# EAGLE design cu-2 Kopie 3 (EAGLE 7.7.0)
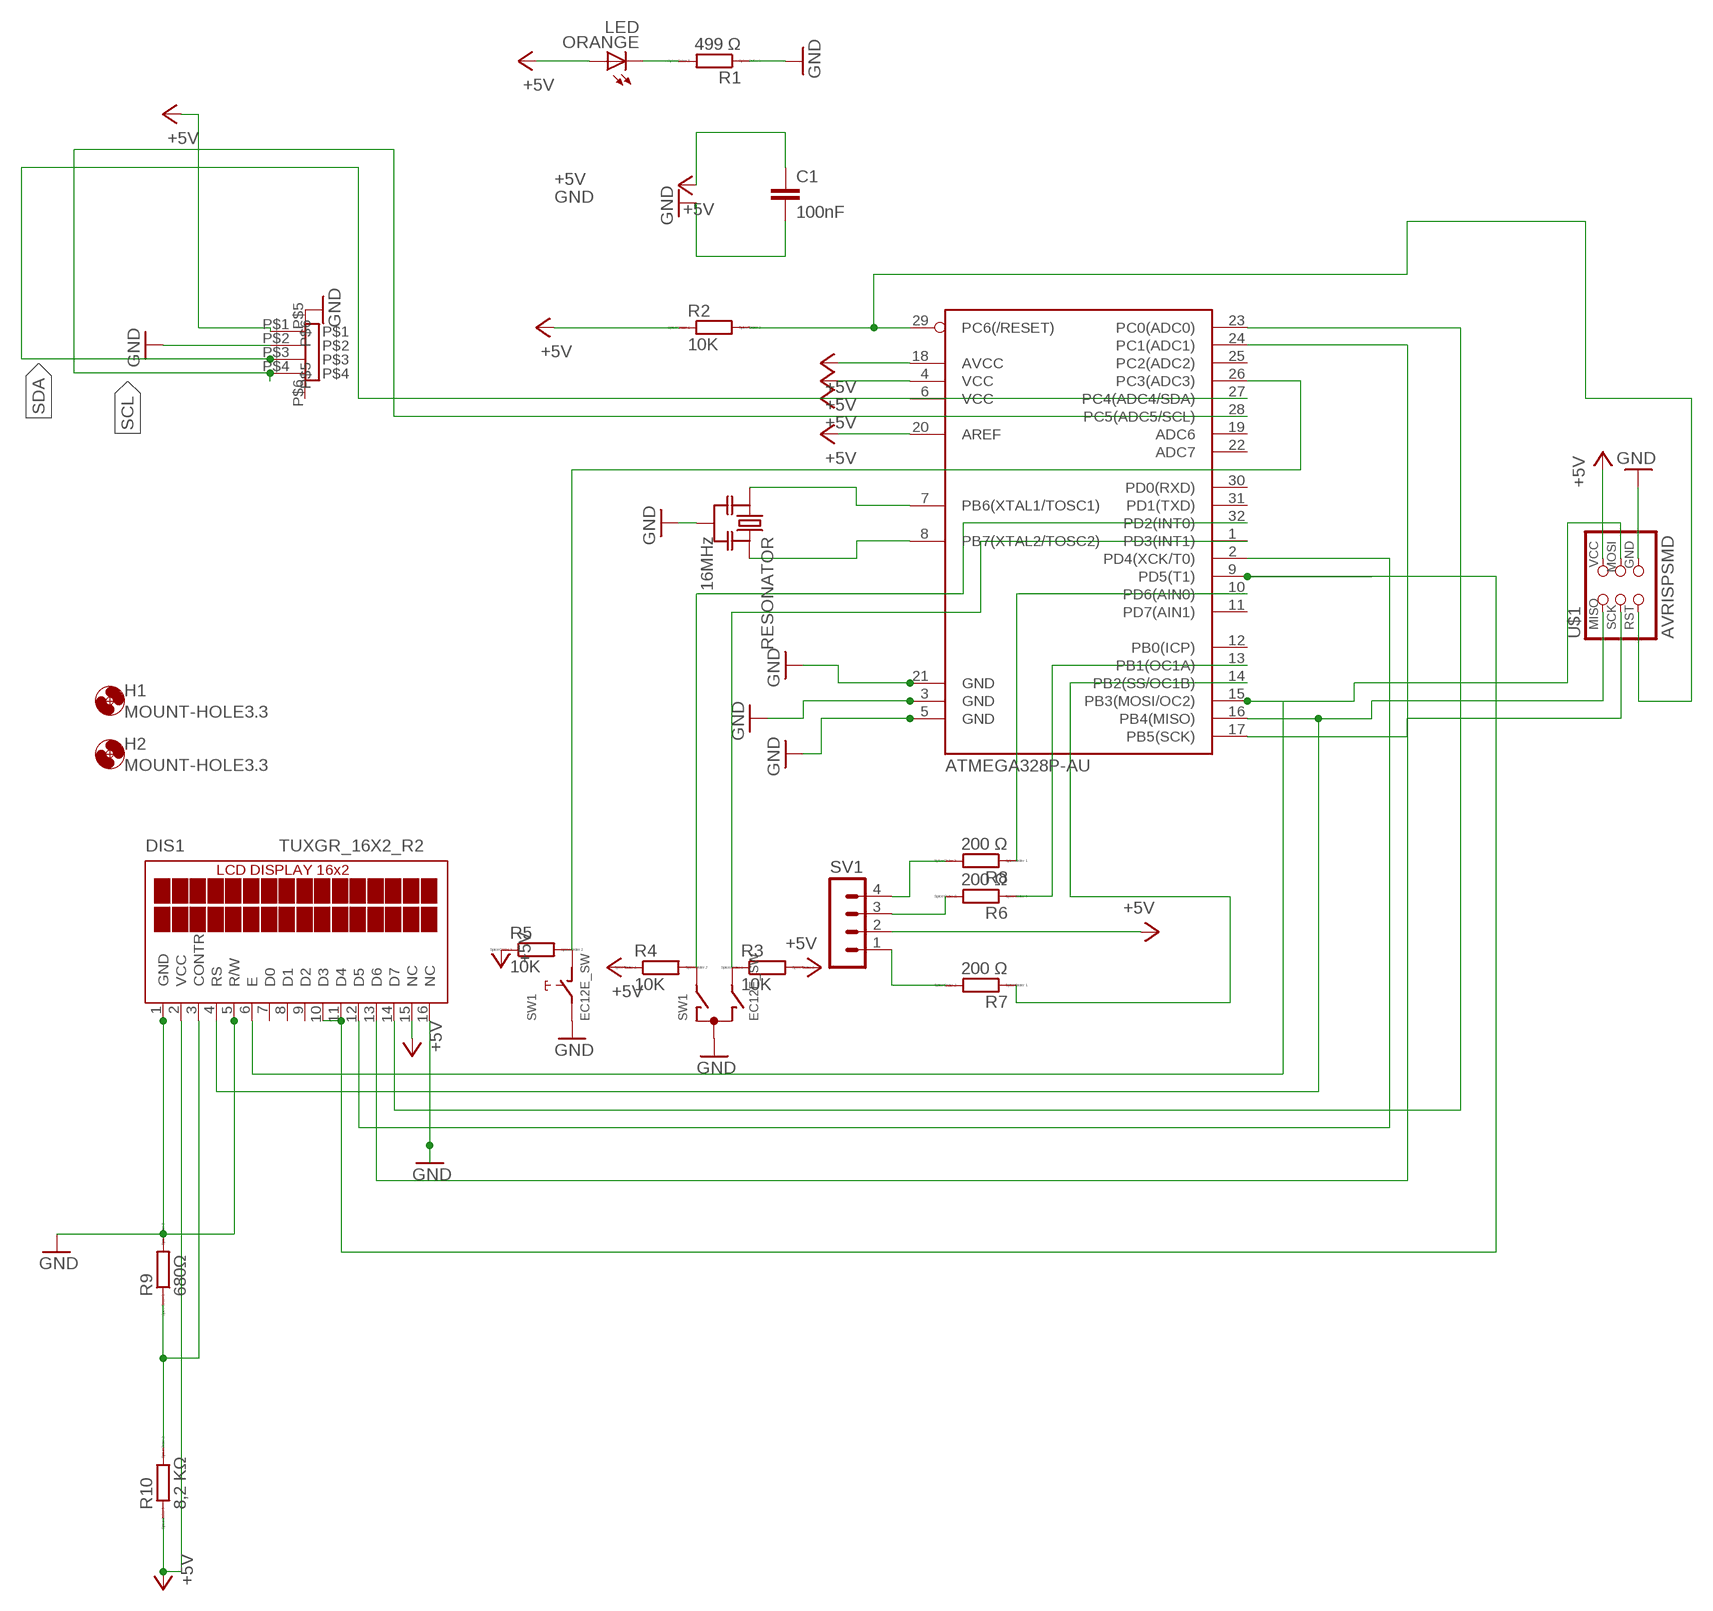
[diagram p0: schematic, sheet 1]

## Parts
ATMEGA328P-AU  ATMEGA88-THIN  [TQFP32-08THIN]
C1  100nF  C-EUC1206  [C1206]
DIS1  TUXGR_16X2_R2  [TUXGR_16X2_R2]
H1  MOUNT-HOLE3.3  [3,3]
H2  MOUNT-HOLE3.3  [3,3]
ORANGE  LED  [LED1206]
R1  499 Ω  RR1206  [R1206]
R2  10K  RR1206  [R1206]
R3  10K  RR1206  [R1206]
R4  10K  RR1206  [R1206]
R5  10K  RR1206  [R1206]
R6  200 Ω  RR1206  [R1206]
R7  200 Ω  RR1206  [R1206]
R8  200 Ω  RR1206  [R1206]
R9  680Ω  RR1206  [R1206]
R10  8,2 KΩ  RR1206  [R1206]
RESONATOR  16MHz  RESONATOR-MURATACSTCR_G  [RESONATOR_MURATA3]
SV1  MA04-1  [MA04-1]
SW1  EC12E_SW  [ALPS_EC12E_SW]
U$1  AVRISPSMD  [2X03SMD]
U$2  PHP4_SM4  [PH4P_SM4]

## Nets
+5V: ATMEGA328P-AU.4(VCC) ATMEGA328P-AU.6(VCC) ATMEGA328P-AU.18(AVCC) ATMEGA328P-AU.20(AREF) C1.1 DIS1.2(VCC) DIS1.15(NC) ORANGE.1(A) R2.1 R3.2 R4.1 R5.1 R10.1 SV1.2 U$1.2(VCC) U$2.P$1
DISP_D4: ATMEGA328P-AU.9(PD5(T1)) DIS1.11(D4)
DISP_D5: ATMEGA328P-AU.2(PD4(XCK/T0)) DIS1.12(D5)
DISP_D6: ATMEGA328P-AU.24(PC1(ADC1)) DIS1.13(D6)
DISP_D7: ATMEGA328P-AU.23(PC0(ADC0)) DIS1.14(D7)
ENC_A: ATMEGA328P-AU.32(PD2(INT0)) R4.2 SW1.A
ENC_B: ATMEGA328P-AU.1(PD3(INT1)) R3.1 SW1.B
GND: ATMEGA328P-AU.3(GND) ATMEGA328P-AU.5(GND) ATMEGA328P-AU.21(GND) C1.2 DIS1.1(GND) DIS1.5(R/W) DIS1.16(NC) R1.1 R9.2 RESONATOR.2 SW1.C SW1.E U$1.6(GND) U$2.P$2 U$2.P$5
N$3: ATMEGA328P-AU.26(PC3(ADC3)) R5.2 SW1.D
N$4: ATMEGA328P-AU.10(PD6(AIN0)) R8.1
N$6: ATMEGA328P-AU.15(PB3(MOSI/OC2)) DIS1.6(E) U$1.4(MOSI)
N$10: DIS1.3(CONTR) R9.1 R10.2
N$11: ATMEGA328P-AU.13(PB1(OC1A)) R6.1
N$12: ATMEGA328P-AU.14(PB2(SS/OC1B)) R7.1
N$13: R7.2 SV1.1
N$14: R6.2 SV1.3
N$15: R8.2 SV1.4
N$19: ATMEGA328P-AU.17(PB5(SCK)) U$1.3(SCK)
N$20: ATMEGA328P-AU.16(PB4(MISO)) DIS1.4(RS) U$1.1(MISO)
N$24: ORANGE.2(C) R1.2
N$27: ATMEGA328P-AU.7(PB6(XTAL1/TOSC1)) RESONATOR.1
N$28: ATMEGA328P-AU.8(PB7(XTAL2/TOSC2)) RESONATOR.3
N$29: ATMEGA328P-AU.29(PC6(/RESET)) R2.2 U$1.5(RST)
SCL: ATMEGA328P-AU.28(PC5(ADC5/SCL)) U$2.P$4
SDA: ATMEGA328P-AU.27(PC4(ADC4/SDA)) U$2.P$3
Unconnected: ATMEGA328P-AU.11(PD7(AIN1)) ATMEGA328P-AU.12(PB0(ICP)) ATMEGA328P-AU.19(ADC6) ATMEGA328P-AU.22(ADC7) ATMEGA328P-AU.25(PC2(ADC2)) ATMEGA328P-AU.30(PD0(RXD)) ATMEGA328P-AU.31(PD1(TXD)) DIS1.7(D0) DIS1.8(D1) DIS1.9(D2) DIS1.10(D3) SW1.GND1(G) SW1.GND2(G) U$2.P$6

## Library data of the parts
ATMEGA328P-AU = fab:ATMEGA88-THIN
C1 = rcl:C-EU: CAPACITOR, European symbol
DIS1 = display-lcd:TUXGR_16X2_R2: Tuxgraphics LCD display 16x2 characters reflective, without background light Source: tuxgr_12x2_r2.pdf; OC_FARNELL: unknown; OC_NEWARK: unknown
H1 H2 = holes:MOUNT-HOLE: MOUNTING HOLE with drill center marker
ORANGE = fab:LED: LED
R1-R10 = eagle-ltspice:R: RESISTOR, European symbol; SPICEMODEL: NONE; SPICEPREFIX: R
RESONATOR = m-pad-2.1:RESONATOR-MURATA: Murata ceramic Resonator "ceralock" CSTCE series with built in load capacitance +- 0.5% tolerance 12.51MHz to 19.99MHz 16MHz murata part#: CSTCE16M0V53-R0 16MHz digikey part#: 490-1198-1-ND $1.33 each
SV1 = con-lstb:MA04-1: PIN HEADER; OC_FARNELL: unknown; OC_NEWARK: unknown
SW1 = switch-alps:EC12E_SW: ALPS rotary Encoder EC12E series with switch; MPN: EC12E2424407; OC_FARNELL: 1520813; OC_NEWARK: 74M1068
U$1 = fab:AVRISP
U$2 = jst_ph_topo:PHP4_SM4

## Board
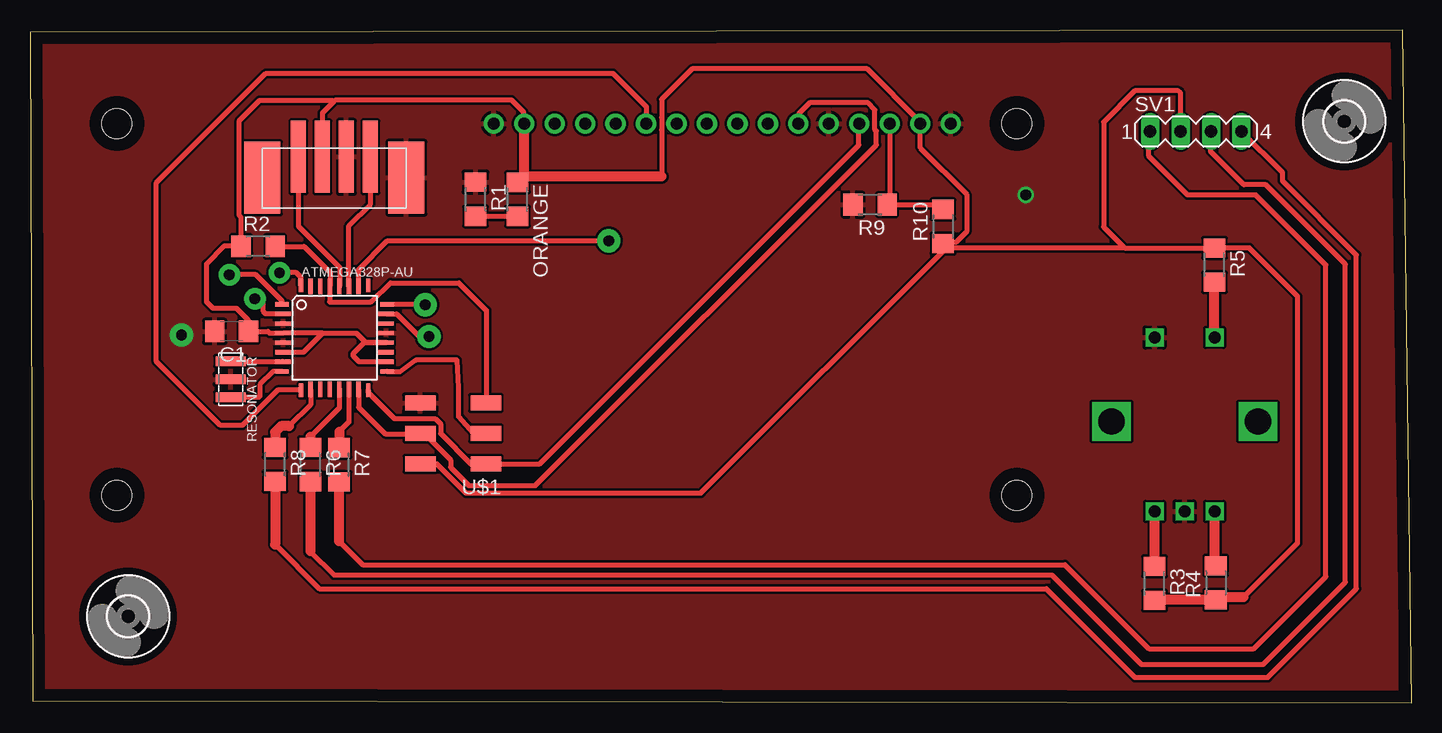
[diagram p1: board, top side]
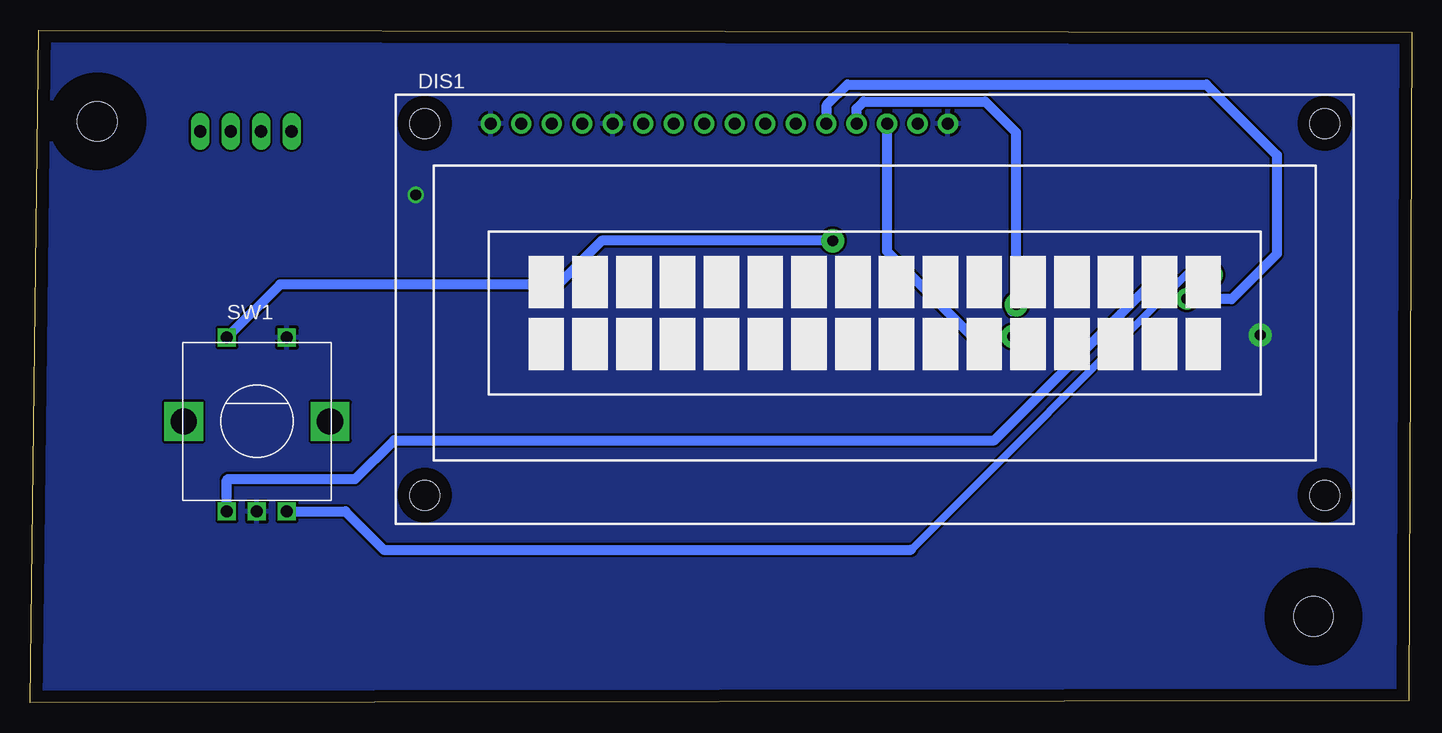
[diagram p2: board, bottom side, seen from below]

Size 115.13 x 56.12 mm. Coordinates in mm from the lower left corner, seen from the top.
Outline: 0.24,0.18 115.13,0 114.39,56.12 0,55.91 0.24,0.18
Copper layers (1*16): Top 0.035mm / dielectric 1.5mm / Bottom 0.035mm
Design rules "default": minimum track width 10mil, minimum drill 24mil, track to track 8mil, track to pad 8mil, pad to pad 8mil, via to via 8mil, smd to smd 8mil, copper to edge 40mil, drill to drill 8mil, minimum pad ring 10mil, minimum via ring 8mil, stop-mask expansion 4mil, vias tented up to drill 0mil, thermal gap 10mil

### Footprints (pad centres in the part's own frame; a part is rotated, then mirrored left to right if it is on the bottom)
TQFP32-08THIN = smd 1.118 x 0.356: 1 -4.369,2.8; 8 -4.369,-2.8; 17 4.369,-2.8; 24 4.369,2.8 | smd 1.27 x 0.356: 2 -4.293,2; 3 -4.293,1.2; 4 -4.293,0.4; 5 -4.293,-0.4; 6 -4.293,-1.2; 7 -4.293,-2; 18 4.293,-2; 19 4.293,-1.2; 20 4.293,-0.4; 21 4.293,0.4; 22 4.293,1.2; 23 4.293,2 | smd 0.356 x 1.118: 9 -2.8,-4.369; 16 2.8,-4.369; 25 2.8,4.369; 32 -2.8,4.369 | smd 0.356 x 1.27: 10 -2,-4.293; 14 1.2,-4.293; 15 2,-4.293; 26 2,4.293; 27 1.2,4.293; 31 -2,4.293 | smd 0.35 x 1.27: 11 -1.2,-4.293; 12 -0.4,-4.293; 13 0.4,-4.293; 28 0.4,4.293; 29 -0.4,4.293; 30 -1.2,4.293
C1206 = smd 1.6 x 1.8: 1 -1.4,0; 2 1.4,0
TUXGR_16X2_R2 = drill 1 pad 1.676: 1 -32,15.5; 2 -29.46,15.5; 3 -26.92,15.5; 4 -24.38,15.5; 5 -21.84,15.5; 6 -19.3,15.5; 7 -16.76,15.5; 8 -14.22,15.5; 9 -11.68,15.5; 10 -9.14,15.5; 11 -6.6,15.5; 12 -4.06,15.5; 13 -1.52,15.5; 14 1.02,15.5; 15 3.56,15.5; 16 6.1,15.5 | hole 2.5: -37.5,-15.5; 37.5,-15.5; -37.5,15.5; 37.5,15.5
3,3 = hole 3.3: 0,0
LED1206 = smd 1.6 x 1.803: 1 -1.422,0; 2 1.422,0
R1206 = smd 1.6 x 1.803: 1 -1.422,0; 2 1.422,0
RESONATOR_MURATA3 = smd 0.8 x 2.5: 1 -1.5,0; 2 0,0; 3 1.5,0
MA04-1 = drill 1.016 long: 1 -3.81,0; 2 -1.27,0; 3 1.27,0; 4 3.81,0
ALPS_EC12E_SW = drill 1 square: A -2.5,-7.5; B 2.5,-7.5; C 0,-7.5; D -2.5,7; E 2.5,7 | drill 2.2 square: GND1 -6.1,0; GND2 6.1,0
2X03SMD = smd 2.54 x 1.27: 1 -2.54,2.54; 2 2.92,2.54; 3 -2.54,0; 4 2.92,0; 5 -2.54,-2.54; 6 2.92,-2.54
PH4P_SM4 = smd 6 x 1.27: P$1 2,2; P$2 2,4; P$3 2,6; P$4 2,0 | smd 6 x 3: P$5 3.75,9; P$6 3.75,-3

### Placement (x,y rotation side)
ATMEGA328P-AU  25.38,30.44 0 top
C1  16.8,30.98 180 top
DIS1  44.74,32.81 0 bottom
H1  109.52,48.5 0 top
H2  8.18,7.22 0 top
ORANGE  40.62,41.99 270 top
R1  37.13,42 270 top
R2  19.01,38.06 0 top
R3  93.7,9.96 270 top
R4  98.82,10.02 90 top
R5  98.71,36.51 270 top
R6  23.37,19.88 270 top
R7  25.75,19.86 270 top
R8  20.42,19.89 270 top
R9  70,41.55 180 top
R10  76.08,39.73 90 top
RESONATOR  16.72,26.99 270 top
SV1  97.15,47.65 0 top
SW1  96.22,23.47 0 bottom
U$1  35.46,22.47 180 top
U$2  22.36,47.55 270 top

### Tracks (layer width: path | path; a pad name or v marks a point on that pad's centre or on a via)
+5V
  Top 0.406: U$2.P$1 24.36,49.2 25.3,50.14 | 25.3,50.14 25.45,50.28 40.12,50.28 41.11,49.29 41.11,48.38 DIS1.15 | ORANGE.1 41.18,43.97 41.25,43.89 | R2.1 17.58,40.5 17.46,40.63 17.46,48.56 19.14,50.25 25.19,50.25 25.3,50.14 | 18.2,37.45 R2.1 | 24.41,30.84 ATMEGA328P-AU.4 21.07,30.83 19.98,30.83 19.83,30.98 C1.1 18.2,31.92 17.23,32.89 15.27,32.89 14.72,33.44 14.72,36.61 16.22,38.12 17.53,38.12 R2.1 | 24.41,30.84 27.2,30.84 27.97,30.07 29.65,30.07 ATMEGA328P-AU.20 27.85,30.04 26.93,29.12 26.93,28.95 27.41,28.46 29.66,28.46 ATMEGA328P-AU.18 | ATMEGA328P-AU.6 22.81,29.24 24.41,30.84 | 76.19,38.42 77.17,38.42 78.05,39.3 78.05,42.42 74.2,46.28 DIS1.2 74.2,48.43 69.76,52.87 55.18,52.87 52.64,50.33 52.64,48.84 52.63,48.83 52.63,47.8 52.64,47.79 52.64,43.89 | R10.1 76.19,38.42 | 93.44,8.6 93.17,8.32 93.48,8.32 R3.2 | 101.12,8.81 105.62,13.31 105.62,33.93 101.62,37.93 R5.1 91.23,37.93 | 99.03,8.81 R4.1 | 91.23,37.93 76.68,37.93 76.5,38.11 | 76.5,38.11 76.19,38.42 | U$1.2 33.9,19.93 36.32,17.51 55.9,17.51 76.5,38.11 | SV1.2 95.88,50.87 95.69,51.05 92.08,51.05 89.47,48.44 89.47,39.7 91.23,37.93
  Top 0.813: 41.18,43.97 DIS1.15 | R4.1 93.44,8.6 | 101.12,8.81 99.03,8.81 | 52.64,43.89 41.25,43.89
DISP_D4
  Top 0.406: ATMEGA328P-AU.9 20.63,26.08 17.7,23.14 15.87,23.14 10.54,28.47 10.54,43.38 19.67,52.51 48.57,52.51 51.36,49.72 51.36,48.34 DIS1.11
DISP_D5  (via drill 0.9 pad 1.78)
  Top 0.406: ATMEGA328P-AU.2 19.64,32.44 19.44,32.64 19.44,33.62 v18.74,33.7
  Bottom 0.406: 19.44,33.61 v18.74,33.7 | 48.73,48.24 DIS1.12
  Bottom 0.813: 48.73,48.24 48.73,49.87 47.03,51.57 17.1,51.57 11.22,45.69 11.22,37.44 15.01,33.66 18.7,33.66 v18.74,33.7
DISP_D6  (via drill 0.9 pad 1.93)
  Top 0.406: ATMEGA328P-AU.24 32.91,33.24 v32.95,33.2
  Bottom 0.813: DIS1.13 46.26,49.57 45.67,50.15 35.54,50.15 32.97,47.58 32.97,32.99 33.31,32.65 33.31,32.84 v32.95,33.2
DISP_D7  (via drill 0.9 pad 1.93)
  Top 0.406: ATMEGA328P-AU.23 30.55,32.44 32.49,30.5 33.18,30.5 v33.25,30.56
  Bottom 0.813: v33.25,30.56 36.63,30.56 43.72,37.65 DIS1.14
ENC_A  (via drill 0.9 pad 1.78)
  Top 0.406: 98.72,11.53 R4.2 | ATMEGA328P-AU.32 22.58,35.5 22.21,35.87 v20.79,35.87
  Top 0.813: 98.72,11.53 SW1.A
  Bottom 0.813: SW1.A 98.72,18.58 98.64,18.66 88.03,18.66 84.79,21.9 34.76,21.9 v20.79,35.87
ENC_B  (via drill 0.9 pad 1.78)
  Top 0.406: 93.72,11.4 R3.1 | ATMEGA328P-AU.1 21.01,33.52 18.83,35.7 v16.62,35.7
  Top 0.813: 93.72,11.4 SW1.B
  Bottom 0.61: 41.7,12.78 18.74,35.75 16.66,35.75
  Bottom 0.813: SW1.B 88.86,15.97 85.67,12.78 41.7,12.78 | 16.66,35.75 v16.62,35.7
GND  (via drill 0.9 pad 1.2, 0.9 pad 1.93)
  other vias: 12.62,30.69 82.98,42.36
  pour Top: 114.27,140.93 -28.96,140.1 -30.36,-28.63 113.76,-26.08
  pour Bottom: 122.38,64.58 136.04,52.69 136.04,6.39 120.7,-8.95 -13.54,-8.95 -21.13,-1.36 -20.99,65.48
N$3  (via drill 0.9 pad 1.93)
  Top 0.406: 98.71,30.49 SW1.D | ATMEGA328P-AU.26 27.38,36.14 29.79,38.55 48.22,38.55 v48.23,38.54
  Top 0.813: 98.71,30.49 R5.2
  Bottom 0.813: v48.23,38.54 67.49,38.54 71.13,34.9 94.29,34.9 SW1.D
N$4
  Top 0.406: ATMEGA328P-AU.10 23.38,24.86 21.59,23.08 | 20.43,21.32 R8.1
  Top 0.813: 21.59,23.08 20.92,23.08 20.43,22.59 20.43,21.32
N$6
  Top 0.406: ATMEGA328P-AU.15 27.38,24.65 29.6,22.43 33.33,22.43 32.57,22.43 U$1.4 32.84,22.47 35.05,20.25 35.05,19.64 36.58,18.12 42.12,18.12 70.53,46.52 70.53,47.68 70.41,47.8 70.41,49.47 69.85,50.03 64.97,50.03 64.03,49.09 64.03,48.32 DIS1.6
N$10
  Top 0.406: DIS1.3 71.66,41.79 R9.1 75.68,41.56 R10.2
N$11
  Top 0.406: ATMEGA328P-AU.13 25.78,24.61 23.37,22.19 | R6.1
  Top 0.813: 23.37,22.19 R6.1
N$12
  Top 0.406: ATMEGA328P-AU.14 26.58,23.42 25.78,22.62 | 25.78,21.31 R7.1
  Top 0.813: 25.78,22.62 25.78,21.31
N$13
  Top 0.406: 25.75,13.49 27.72,11.52 86.23,11.52 93.23,4.52 102,4.52 108,10.52 108,36.52 102.15,42.36 96.46,42.36 93.23,45.59 93.23,47.55 SV1.1
  Top 0.813: R7.2 25.75,13.49
N$14
  Top 0.406: 23.37,12.65 25.34,10.67 85.16,10.67 92.62,3.21 102.77,3.21 109.61,10.06 109.61,36.59 103,43.21 101.15,43.21 98.38,45.98 98.38,47.62 SV1.3
  Top 0.813: R6.2 23.37,12.65
N$15
  Top 0.406: 20.42,13.21 24.11,9.52 84.7,9.52 92.08,2.13 103.15,2.13 110.53,9.52 110.53,37.36 104.38,43.51 104.38,44.23 SV1.4
  Top 0.813: R8.2 20.42,13.21
N$19
  Top 0.406: U$1.3 36.99,22.47 35.71,23.87 35.71,26.25 35.59,28.58 32.17,28.58 30.82,27.6 29.79,27.6 ATMEGA328P-AU.17
N$20
  Top 0.406: ATMEGA328P-AU.16 28.18,25.9 30.36,23.72 33.77,23.72 34.21,23.27 34.21,22.46 36.75,19.93 U$1.1 | U$1.1 | U$1.1 42.49,19.93 69.08,46.52 69.08,48.28 DIS1.4
N$24
  Top 0.406: ORANGE.2 37.14,40.57 R1.2
N$27
  Top 0.406: RESONATOR.1 21.04,28.49 ATMEGA328P-AU.7
N$28
  Top 0.406: ATMEGA328P-AU.8 20.27,27.64 19.16,26.53 19.16,25.58 19.07,25.49 RESONATOR.3
N$29
  Top 0.406: R2.2 22.85,38.06 25.01,35.9 25.01,34.77 ATMEGA328P-AU.29 24.98,33.46 24.95,33.44 28.41,33.44 28.47,33.5 28.5,33.5 30.03,35.03 35.74,35.03 38.03,32.73 38.03,25.04 U$1.5
SCL
  Top 0.406: U$2.P$4 22.36,39.75 25.81,36.31 25.81,34.77 ATMEGA328P-AU.28
SDA
  Top 0.406: ATMEGA328P-AU.27 26.58,39.8 28.38,41.6 28.38,45.54 U$2.P$3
